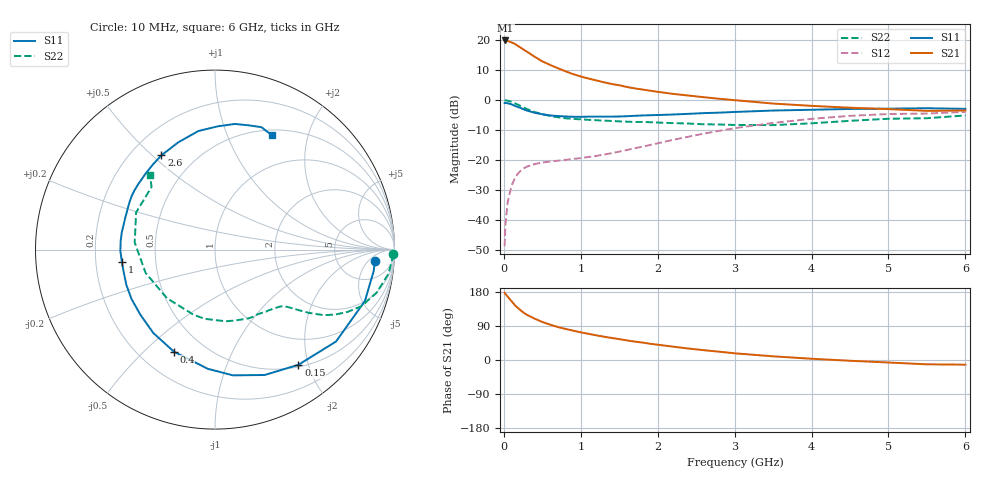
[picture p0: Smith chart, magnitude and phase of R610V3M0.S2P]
! SIEMENS Small Signal Semiconductors
! BFR193
! Si NPN RF Bipolar Junction Transistor in SOT23
! VCE = 10 V  IC = 3 mA
! Common Emitter S-Parameters:  May  1996
# GHz  S  MA  R  50
!  f  S11  S21  S12  S22
! GHz  MAG  ANG  MAG  ANG  MAG  ANG  MAG  ANG
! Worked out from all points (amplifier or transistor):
!   36 points, 10 MHz to 6 GHz, reference 50 ohm
!   highest |S21| = 19.9 dB at 20 MHz (marker M1)
!   |S21| within 3 dB of that: start of sweep to 253.4 MHz
!   unconditionally stable (mu >= 1): 1.086 GHz to 2.046 GHz
!   at 250 MHz: K = 0.30, MSG = 20.0 dB, |S12| = -23.0 dB
!   at 1.4 GHz: K = 1.09, MAG = 9.8 dB, |S12| = -17.8 dB
!   at 6 GHz: K = 0.98, MSG = 0.2 dB, |S12| = -4.0 dB
!   S11 on the Smith chart (normalised r, x): 10 MHz: 13, -8; 150 MHz: 0.53, -1.84; 400 MHz: 0.34, -0.62; 1 GHz: 0.31, -0.06; 2.6 GHz: 0.32, +0.54; 6 GHz: 0.56, +1.46
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0.01  0.8937 -4.0  9.762 177.6  0.0036 84.9  0.9939 -1.5
0.02  0.8921 -7.7  9.909 174.5  0.0081 81.9  0.9882 -3.2
0.05  0.883 -18.9  9.712 167.1  0.0196 79.3  0.9763 -7.9
0.1  0.8468 -37.2  9.195 155.1  0.0369 70.1  0.9323 -14.9
0.15  0.7924 -54.1  8.59 143.2  0.0515 62.5  0.8749 -21.1
0.2  0.7514 -68.4  7.783 134.3  0.0624 56.3  0.8159 -25.2
0.25  0.7076 -81.9  7.06 125.9  0.0711 51.4  0.759 -28.5
0.3  0.6656 -93.4  6.429 119.2  0.0769 48.1  0.707 -31.1
0.4  0.6129 -112.0  5.298 109.1  0.0848 43.3  0.6305 -34.0
0.5  0.5779 -126.5  4.429 100.4  0.0902 40.6  0.5803 -35.7
0.6  0.5518 -138.9  3.871 93.4  0.0937 40.1  0.5431 -37.1
0.7  0.5404 -149.4  3.413 87.2  0.0968 40.8  0.5157 -38.3
0.8  0.5317 -158.1  3.03 82.1  0.0998 41.7  0.4959 -39.6
1  0.5233 -172.3  2.475 73.0  0.1069 45.2  0.4757 -42.4
1.1  0.5273 -179.2  2.288 69.1  0.1114 47.1  0.4664 -44.5
1.6  0.5362 155.5  1.653 51.7  0.1461 57.2  0.4342 -55.6
2.2  0.5726 132.8  1.266 35.2  0.2158 60.9  0.4113 -73.6
2.6  0.6042 119.6  1.114 25.9  0.2742 58.5  0.3932 -89.2
3.5  0.6671 98.0  0.873 9.7  0.4139 45.6  0.3807 -134.5
4.5  0.7088 81.0  0.743 -2.0  0.5437 27.0  0.4492 174.9
5.5  0.7295 69.2  0.659 -11.4  0.5948 8.3  0.4963 135.4
6  0.7119 63.7  0.667 -12.3  0.6321 3.0  0.5525 131.0
